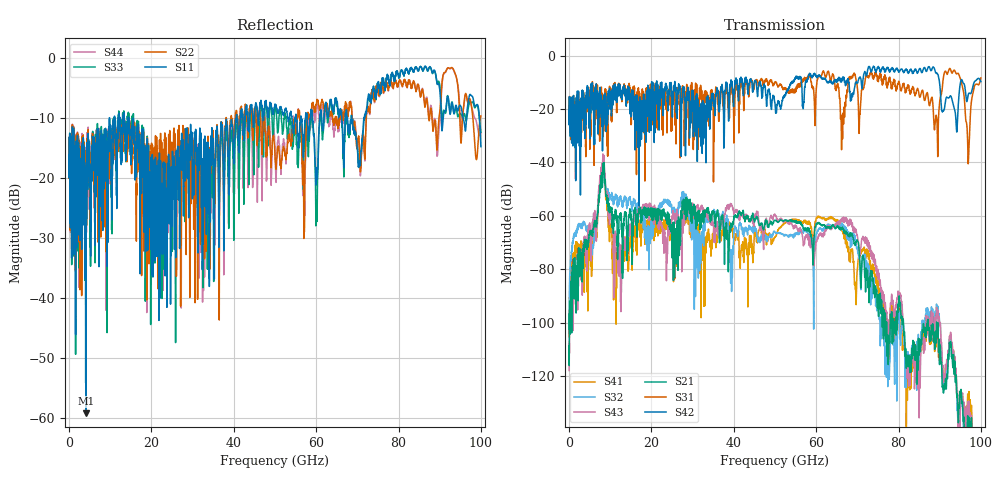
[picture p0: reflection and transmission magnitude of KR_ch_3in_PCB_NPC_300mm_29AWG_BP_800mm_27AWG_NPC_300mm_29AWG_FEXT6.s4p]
# GHz S RI R 45
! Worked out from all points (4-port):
!   4000 points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, 25 MHz to 100 GHz, reference 45 ohm
!   strongest paths, dB at 25 MHz, 25.02 GHz, 50.02 GHz, 75.03 GHz, 100 GHz:
!     S42: -20.6, -18.0, -18.0, -4.3, -9.8
!     S31: -20.6, -21.5, -10.2, -8.8, -8.4
!     S21: -108.7, -70.3, -61.7, -91.6, -164.3
!     S43: -117.9, -60.8, -59.6, -81.9, -159.1
!     S32: -98.4, -58.7, -66.1, -95.5, -174.7
!     S41: -105.3, -67.6, -68.1, -85.5, -158.2
!   lowest |S11| = -59.2 dB at 4.075 GHz (marker M1), VSWR 1.00, Z = 45 - j0.099 ohm
!   |S11| at or under -10 dB: start of sweep to 9.824 GHz; 14.45 GHz to 40.62 GHz (26.16 GHz wide, 95 % of centre); 68.66 GHz to 71.57 GHz (2.914 GHz wide, 4.16 % of centre)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
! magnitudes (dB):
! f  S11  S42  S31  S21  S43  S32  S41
! 25 MHz  -16.1  -20.6  -20.6  -108.7  -117.9  -98.4  -105.3
! 4.075 GHz  -59.2  -25.8  -37.9  -69.3  -70.1  -64.6  -72.9
! 8.2 GHz  -17.8  -26.6  -22.6  -42.3  -38.4  -40.8  -39.8
! 12.32 GHz  -10.7  -12.6  -12.2  -60.0  -75.9  -53.2  -76.2
! 39.1 GHz  -12.4  -10.9  -13.2  -65.5  -56.0  -73.7  -64.2
! 96.88 GHz  -7.5  -15.0  -38.3  -139.4  -134.7  -144.0  -131.0
! 100 GHz  -14.8  -9.8  -8.4  -164.3  -159.1  -174.7  -158.2
